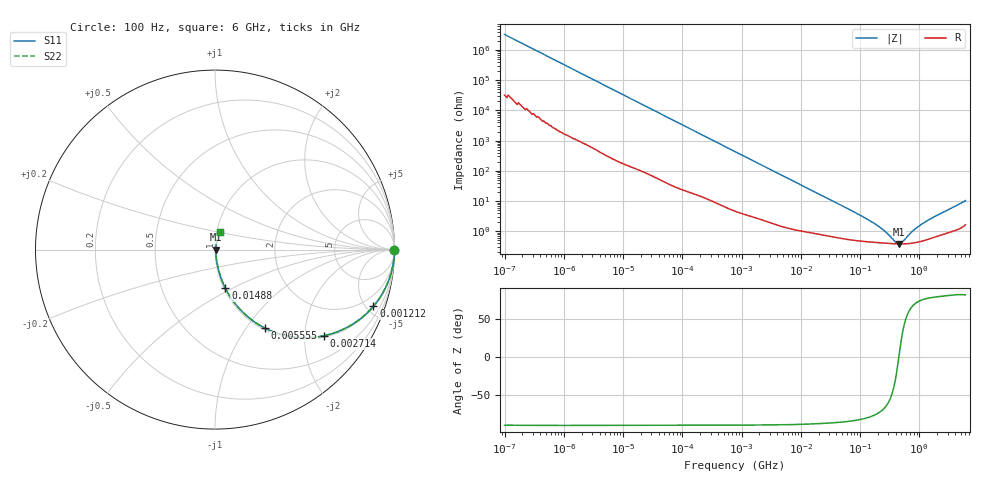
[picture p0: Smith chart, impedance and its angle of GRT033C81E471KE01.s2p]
!Murata Part Number: GRT033C81E471KE01
!These Parameters are Measured in Series Mode Connection
!Data Generated on Jun 19, 2026
!  o--ll--o
!Port1  Port2
!  o------o
!Operation Temp=25[degC], DC Bias Voltage=0[V]
!Freq. Start=100[Hz] Stop=6[GHz] 401[Steps]
# Hz S RI R 50
!Freq.(Hz) S11(Real) S11(Imag) S21(Real) S21(Imag) S12(Real) S12(Imag) S22(Real) S22(Imag)
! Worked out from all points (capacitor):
!   401 points, 100 Hz to 6 GHz, reference 50 ohm
!   read as one part in series: C = 489 pF near 109 Hz
!   lowest |Z| = 385 mohm at 447 MHz (marker M1)
!   series resonance near 452.3 MHz, so ESL is about 250 pH
!   S11 on the Smith chart (normalised r, x): 100 Hz: open; 1.212 MHz: 1.07, -5.56; 2.714 MHz: 1.04, -2.50; 5.555 MHz: 1.03, -1.23; 14.88 MHz: 1.02, -0.46; 6 GHz: 1.03, +0.20
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100  1 -3.08e-05  3e-07 3.08e-05  3e-07 3.08e-05  1 -3.08e-05
335  1 -0.000103  7e-07 0.000103  7e-07 0.000103  1 -0.000103
2008  1 -0.000612  3.6e-06 0.000612  3.6e-06 0.000612  1 -0.000612
40335  0.9998 -0.0122  0.000226 0.0122  0.000226 0.0122  0.9998 -0.0122
241822  0.9941 -0.0719  0.00586 0.0719  0.00586 0.0719  0.9941 -0.0719
774597  0.9476 -0.2176  0.0524 0.2176  0.0524 0.2176  0.9476 -0.2176
1212075  0.8826 -0.3158  0.1174 0.3158  0.1174 0.3158  0.8826 -0.3158
2713602  0.6083 -0.4799  0.3917 0.4799  0.3917 0.4799  0.6083 -0.4799
5554849  0.2784 -0.4375  0.7216 0.4375  0.7216 0.4375  0.2784 -0.4375
8692127  0.1412 -0.3348  0.8588 0.3348  0.8588 0.3348  0.1412 -0.3348
1.487547e7  0.0584 -0.2161  0.9416 0.2161  0.9416 0.2161  0.0584 -0.2161
1.555665e7  0.0543 -0.2076  0.9457 0.2076  0.9457 0.2076  0.0543 -0.2076
3.80911e7  0.0144 -0.0895  0.9856 0.0895  0.9856 0.0895  0.0144 -0.0895
1.275994e8  0.00519 -0.0257  0.9948 0.0257  0.9948 0.0257  0.00519 -0.0257
2.183701e8  0.00432 -0.0127  0.9957 0.0127  0.9957 0.0127  0.00432 -0.0127
3.124326e8  0.00399 -0.00613  0.996 0.00613  0.996 0.00613  0.00399 -0.00613
3.908258e8  0.00387 -0.00239  0.9961 0.00239  0.9961 0.00239  0.00387 -0.00239
4.470121e8  0.00383 -0.000189  0.9962 0.000189  0.9962 0.000189  0.00383 -0.000189
5.112761e8  0.00383 0.00203  0.9962 -0.00203  0.9962 -0.00203  0.00383 0.00203
8.000355e8  0.00421 0.00994  0.9958 -0.00994  0.9958 -0.00994  0.00421 0.00994
1.197065e9  0.00526 0.0185  0.9947 -0.0185  0.9947 -0.0185  0.00526 0.0185
6e9  0.0261 0.0979  0.9739 -0.0979  0.9739 -0.0979  0.0261 0.0979
